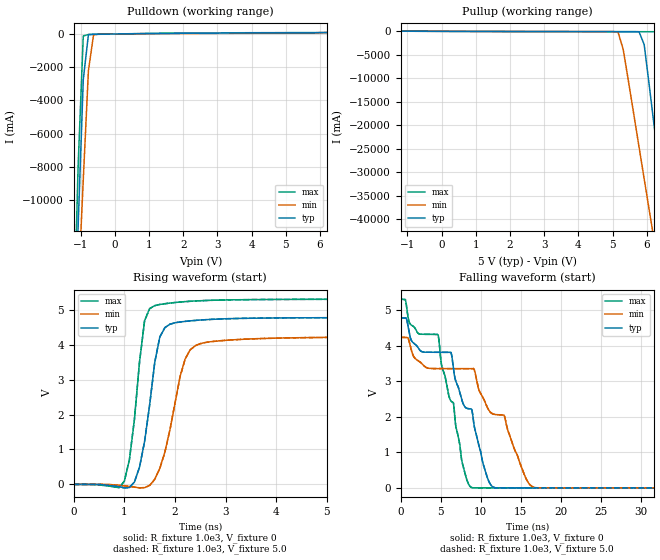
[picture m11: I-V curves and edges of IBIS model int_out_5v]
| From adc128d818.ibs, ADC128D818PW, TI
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[Model] int_out_5v
Model_type Output
Vmeas = 1.4V
Cref = 0.0pF
Rref = 1.0e3
Vref = 0.0V
C_comp   50.0pF   40.8pF   56.8pF
[Voltage Range]   5.0V   4.5V   5.5V
[Temperature Range]   25.0   125.0   -40.0
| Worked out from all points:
|   slope of the pulldown table from 0 to 0.75 V, typ, clamps not added: 38.1 ohm
|   slope of the pullup table from 0 to 0.75 V, typ, clamps not added: 46.3 ohm
|   rising waveform, R_fixture 1.0e3, V_fixture 0: 20-80 % time 283ps typ, 376ps min, 232ps max; typ from 0 V to 4.78 V
|   falling waveform, R_fixture 1.0e3, V_fixture 0: 20-80 % time 7.33ns typ, 11.5ns min, 2.74ns max; typ from 4.78 V to 0 V
|   rising waveform, R_fixture 1.0e3, V_fixture 5.0: 20-80 % time 283ps typ, 376ps min, 232ps max; typ from 0 V to 4.78 V
|   falling waveform, R_fixture 1.0e3, V_fixture 5.0: 20-80 % time 7.33ns typ, 11.5ns min, 2.74ns max; typ from 4.78 V to 0 V
[Pullup]
-5V       99.31mA    81.34mA    113.2mA
5.155V    -66.49mA   -149.1mA   -80.99mA
5.305V    -67.01mA   -3.774A    -81.83mA
5.77V     -88.96mA   -24.63A    -83.58mA
5.92V     -2.796A    -31.4A     -83.86mA
6.07V     -11.61A    -38.15A    -84.12mA
6.37V     -29.65A    -51.59A    -102.8mA
6.52V     -38.62A    -58.29A    -4.229A
6.67V     -47.56A    -64.97A    -15.57A
6.97V     -65.38A    -78.32A    -38.48A
7.135V    -75.16A    -85.65A    -51.01A
10V       -243.4A    -212A      -265.8A
[Pulldown]
-5V       -243.4A    -190.1A    -303.1A
-1.22V    -20.58A    -22.33A    -19.35A
-1.07V    -11.56A    -15.5A     -7.919A
-920mV    -2.748A    -8.771A    -119.2mA
-770mV    -40.56mA   -2.222A    -29.7mA
-620mV    -17.61mA   -50.73mA   -22.67mA
295mV     8.243mA    5.398mA    11.06mA
6.355V    100.4mA    91.22mA    85.89mA
10V       175.1mA    135.6mA    198.6mA
[Rising Waveform]
R_fixture=1.0e3
V_fixture=0
V_fixture_min=0
V_fixture_max=0
0s        2.008nV    68.39nV    1.655nV
1ns       -99.57mV   -41.72mV   91.91mV
1.1ns     -91.51mV   -56.8mV    705.3mV
1.3ns     495.2mV    -99.33mV   3.506V
1.5ns     2.278V     -28.64mV   5.036V
1.6ns     3.489V     144.7mV    5.121V
1.8ns     4.491V     920.6mV    5.176V
2.2ns     4.671V     3.59V      5.236V
2.6ns     4.718V     4.064V     5.268V
99.95ns   4.782V     4.234V     5.307V
[Falling Waveform]
R_fixture=1.0e3
V_fixture=0
V_fixture_min=0
V_fixture_max=0
0s        4.782V     4.234V     5.307V
2.2ns     3.938V     3.575V     4.345V
4.7ns     3.813V     3.353V     4.299V
6.3ns     3.805V     3.353V     2.437V
7.8ns     2.374V     3.353V     618.8mV
8.9ns     2.198V     3.351V     7.563mV
11.3ns    69.28mV    2.109V     105.1uV
12.9ns    169.3uV    2.049V     93.77uV
16.8ns    117.7uV    6.169mV    80.02uV
99.95ns   -5.428uV   1.86uV     -3.252uV
[Rising Waveform]
R_fixture=1.0e3
V_fixture=5.0
V_fixture_min=4.5
V_fixture_max=5.5
0s        2.008nV    68.39nV    1.655nV
1ns       -99.57mV   -41.72mV   91.91mV
1.1ns     -91.51mV   -56.8mV    705.3mV
1.3ns     495.2mV    -99.33mV   3.506V
1.5ns     2.278V     -28.64mV   5.036V
1.6ns     3.489V     144.7mV    5.121V
1.8ns     4.491V     920.6mV    5.176V
2.2ns     4.671V     3.59V      5.236V
2.6ns     4.718V     4.064V     5.268V
99.95ns   4.782V     4.234V     5.307V
[Falling Waveform]
R_fixture=1.0e3
V_fixture=5.0
V_fixture_min=4.5
V_fixture_max=5.5
0s        4.782V     4.234V     5.307V
2.2ns     3.938V     3.575V     4.345V
4.7ns     3.813V     3.353V     4.299V
6.3ns     3.805V     3.353V     2.437V
7.8ns     2.374V     3.353V     618.8mV
8.9ns     2.198V     3.351V     7.563mV
11.3ns    69.28mV    2.109V     105.1uV
12.9ns    169.3uV    2.049V     93.77uV
16.8ns    117.7uV    6.169mV    80.02uV
99.95ns   -5.428uV   1.86uV     -3.252uV
[Ramp]
R_load = 1.0e3
dV/dt_r   2.86923E0/3E-10   2.540292E0/4E-10   3.184285E0/2E-10
dV/dt_f   2.869232E0/7.3E-9   2.540289E0/1.15E-8   3.184285E0/2.7E-9
